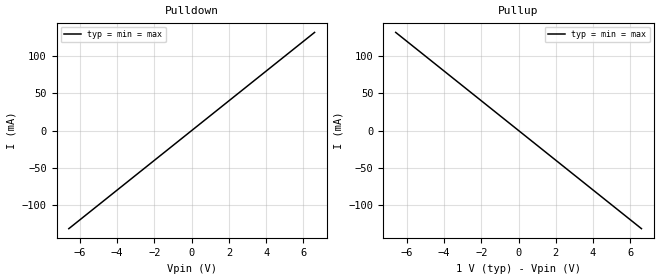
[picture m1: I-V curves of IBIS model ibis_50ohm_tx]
[IBIS Ver]   5.0
[File Name]  TX.ibs
[File Rev]   1.0
[Component]  ibis_50ohm
[Manufacturer] NS
[Package]
R_pkg  0.0   NA   NA
L_pkg  0.0   NA   NA
C_pkg  0.0   NA   NA
[Pin]   signal_name   model_name   R_pin L_pin  C_pin
1p   IBIS_50ohm_Tx_p   ibis_50ohm_tx
1n   IBIS_50ohm_Tx_n   ibis_50ohm_tx
[Diff_Pin] inv_pin vdiff tdelay_typ tdelay_min tdelay_max
1p   1n   NA   NA   NA   NA
| Models and submodels in the file (1): ibis_50ohm_tx (Output)
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[Model] ibis_50ohm_tx
Model_type Output
C_comp 0p 0p 0p
Cref = 0
Vref = 0.5
Rref = 50
Vmeas = 0.5
[Temperature_Range] 25 125 0
[Voltage Range] 1.0 1.0 1.0
[Algorithmic Model]
Executable Windows_VisualC++ExpressEdition9.0.30729_32 IdealTx.dll IdealTx.ami
[End Algorithmic Model]
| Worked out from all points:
|   slope of the pulldown table from 0 to 0.15 V, typ, clamps not added: 50 ohm
|   slope of the pullup table from 0 to 0.15 V, typ, clamps not added: 50 ohm
[Pulldown]
-6.6V     -132mA     -132mA     -132mA
0V        0A         0A         0A
6.6V      132mA      132mA      132mA
[Pullup]
-6.6V     132mA      132mA      132mA
0V        0A         0A         0A
6.6V      -132mA     -132mA     -132mA
[GND Clamp]
-6.6V     0A         0A         0A
0V        0A         0A         0A
6.6V      0A         0A         0A
[Power Clamp]
-6.6V     0A         0A         0A
0V        0A         0A         0A
6.6V      0A         0A         0A
[Ramp]
dV/dt_r 1.0/5p 1.0/5p 1.0/5p
dV/dt_f 1.0/5p 1.0/5p 1.0/5p
